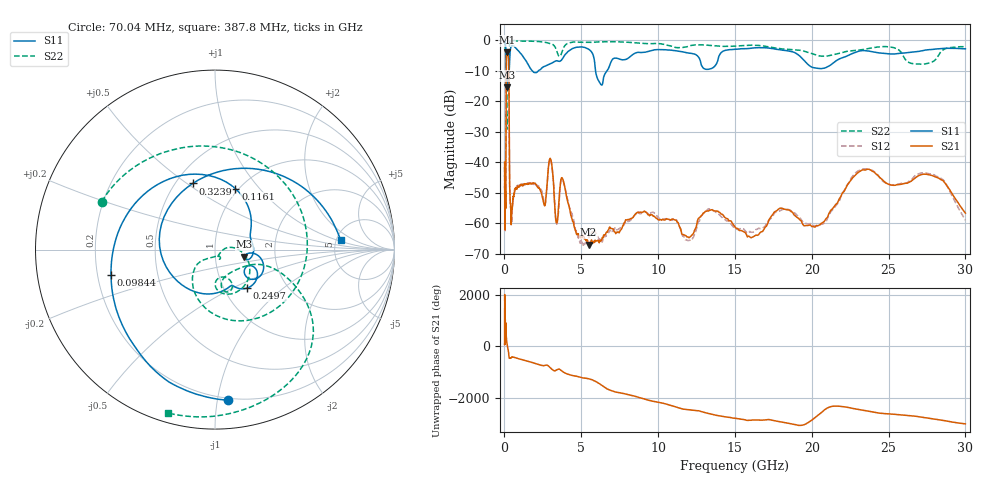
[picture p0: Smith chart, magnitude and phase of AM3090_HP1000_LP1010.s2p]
! Date/Time: Thu, Feb 28, 2019 2:02 PM
! Network Analyzer: Agilent Technologies E8364B Rev: A.07.50.67
! Sweep from 0.010 to 30.000 GHz, 1601 Points, Sweep Type: LOG
! Power Supply: 5.023 V, 0.002 A
# Hz S DB R 50
!freq MagS11 AngS11 MagS21 AngS21 MagS12 AngS12 MagS22 AngS22
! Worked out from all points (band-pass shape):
!   1601 points, 10 MHz to 30 GHz, reference 50 ohm
!   highest |S21| = -4.04 dB at 166.5 MHz (marker M1); lowest = -67.2 dB at 5.473 GHz (marker M2)
!   |S21| within 3 dB of the highest: 122.8 MHz to 273.6 MHz (150.8 MHz wide, 76.1 % of centre)
!   lowest |S11| = -15.5 dB at 153.7 MHz (marker M3), VSWR 1.41, Z = 69.3 - j5.67 ohm
!   |S11| at or under -10 dB: 118.1 MHz to 309.7 MHz (191.6 MHz wide, 89.6 % of centre); 1.793 GHz to 2.229 GHz (436.6 MHz wide, 21.7 % of centre); 5.925 GHz to 6.693 GHz (767.8 MHz wide, 12.2 % of centre)
!   |S22| runs from -29.4 to -0.1 dB; largest |S21 - S12| = 0.017
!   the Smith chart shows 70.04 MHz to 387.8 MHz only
!   S11 on the Smith chart (normalised r, x): 70.04 MHz: 0.19, -1.08; 98.44 MHz: 0.26, -0.11; 116.1 MHz: 0.97, +0.75; 249.7 MHz: 1.27, -0.59; 323.9 MHz: 0.61, +0.53; 387.8 MHz: 5.45, +1.13
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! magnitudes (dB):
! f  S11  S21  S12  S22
! 10 MHz  -0.2  -40.0  -41.9  -0.7
! 38.04 MHz  -0.5  -60.3  -59.7  -1.6
! 70.04 MHz  -1.5  -54.7  -52.8  -3.3
! 98.44 MHz  -4.5  -35.3  -35.3  -5.6
! 116.1 MHz  -8.9  -11.2  -11.2  -10.8
! 144.7 MHz  -14.3  -4.4  -4.4  -29.2
! 153.7 MHz  -15.5  -4.1  -4.1  -24.5
! 166.5 MHz  -13.2  -4.0  -4.0  -15.2
! 249.7 MHz  -11.1  -5.2  -5.2  -12.2
! 285.8 MHz  -12.2  -10.3  -10.2  -11.5
! 323.9 MHz  -8.2  -43.5  -43.7  -1.4
! 387.8 MHz  -3.1  -53.6  -54.0  -0.5
! 550.5 MHz  -1.9  -52.1  -52.8  -0.3
! 2.084 GHz  -10.6  -47.6  -47.6  -0.5
! 2.987 GHz  -7.8  -38.9  -38.9  -1.2
! 3.402 GHz  -6.8  -59.9  -60.4  -3.6
! 3.798 GHz  -6.0  -45.6  -45.9  -3.2
! 5.473 GHz  -3.0  -67.2  -64.9  -0.8
! 7.926 GHz  -6.3  -59.0  -60.0  -0.7
! 16.21 GHz  -2.6  -64.5  -62.9  -1.7
! 23.48 GHz  -3.5  -42.6  -42.3  -3.0
! 30 GHz  -2.9  -56.8  -59.1  -2.2
